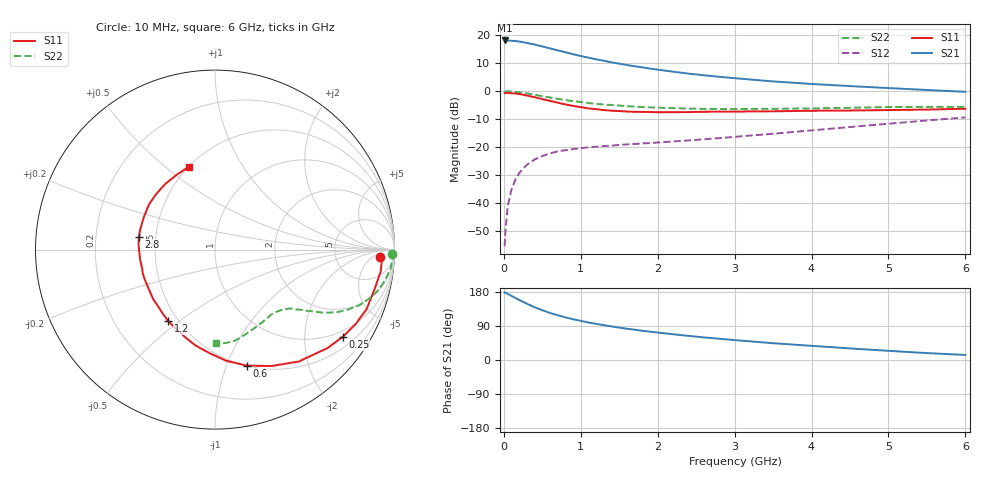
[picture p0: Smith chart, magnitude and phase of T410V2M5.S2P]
! Infineon Technologies  Discrete & RF Semiconductors
! BFR182T
! Si NPN RF Bipolar Junction Transistor in SC75
! VCE = 10 V  IC = 2.5 mA
! Common Emitter S-Parameters:  October  1999
# GHz  S  MA  R  50
!  f  S11  S21  S12  S22
! GHz  MAG  ANG  MAG  ANG  MAG  ANG  MAG  ANG
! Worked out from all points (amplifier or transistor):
!   36 points, 10 MHz to 6 GHz, reference 50 ohm
!   highest |S21| = 18.1 dB at 10 MHz (marker M1)
!   |S21| within 3 dB of that: start of sweep to 622.8 MHz
!   unconditionally stable (mu >= 1): 1.94 GHz to 4.417 GHz
!   at 250 MHz: K = 0.16, MSG = 22.6 dB, |S12| = -27.7 dB
!   at 1.4 GHz: K = 0.81, MSG = 14.9 dB, |S12| = -19.5 dB
!   at 6 GHz: K = 0.84, MSG = 4.6 dB, |S12| = -9.4 dB
!   S11 on the Smith chart (normalised r, x): 10 MHz: 19, -11; 250 MHz: 0.81, -3.05; 600 MHz: 0.50, -1.18; 1.2 GHz: 0.44, -0.46; 2.8 GHz: 0.40, +0.07; 6 GHz: 0.50, +0.61
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0.01  0.923 -2.6  8.043 177.9  0.0017 84.4  0.9864 -1.3
0.02  0.9328 -1.6  8.007 177.9  0.0031 93.6  0.9884 -1.1
0.05  0.9316 -7.4  8.036 174.4  0.0088 86.8  0.9896 -3.1
0.1  0.9163 -13.8  7.948 169.3  0.0175 83.5  0.9844 -6.2
0.2  0.8864 -28.0  7.696 158.4  0.0343 75.5  0.9525 -11.8
0.25  0.862 -34.3  7.489 153.4  0.0412 71.2  0.9321 -14.5
0.3  0.8336 -41.1  7.267 148.4  0.0484 68.2  0.9114 -16.8
0.4  0.7788 -53.2  6.799 139.2  0.0602 62.7  0.862 -21.1
0.5  0.7209 -64.1  6.291 131.4  0.0694 57.8  0.8139 -24.2
0.6  0.67 -74.7  5.799 124.2  0.0774 54.3  0.7701 -26.8
0.8  0.5784 -92.9  4.956 112.5  0.088 49.1  0.6937 -30.4
0.9  0.5453 -101.4  4.571 107.6  0.0923 47.5  0.6615 -31.6
1.1  0.4907 -116.5  3.966 98.9  0.0993 45.4  0.6144 -33.7
1.2  0.4763 -123.3  3.704 95.4  0.1015 44.8  0.5932 -34.5
1.4  0.4471 -135.6  3.27 88.6  0.1062 44.2  0.5649 -36.2
1.6  0.4313 -147.5  2.928 82.5  0.1117 44.7  0.5393 -37.5
2.2  0.4209 -172.3  2.227 67.9  0.1262 48.1  0.4975 -42.8
2.8  0.4299 170.3  1.806 56.1  0.1446 51.8  0.4783 -49.5
3.5  0.4366 154.7  1.492 44.3  0.1733 55.6  0.4835 -57.8
4.5  0.4505 136.8  1.23 30.6  0.2284 57.3  0.5038 -71.0
5.5  0.4686 117.0  1.049 18.2  0.299 55.4  0.524 -83.7
6  0.4848 107.3  0.972 13.4  0.3391 52.9  0.5221 -89.4
